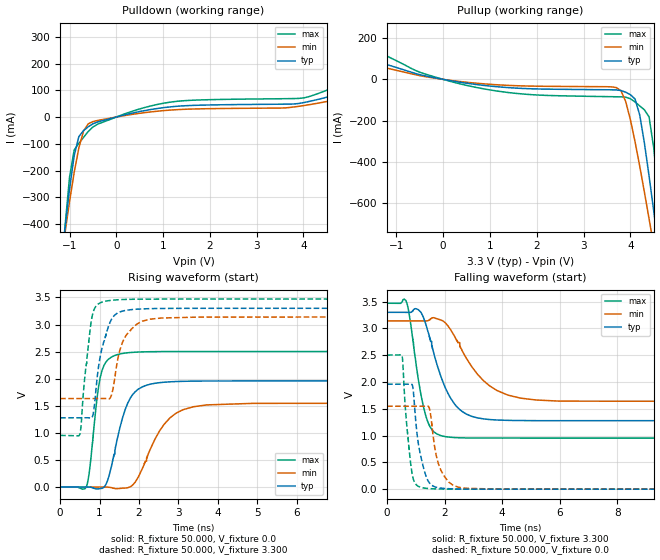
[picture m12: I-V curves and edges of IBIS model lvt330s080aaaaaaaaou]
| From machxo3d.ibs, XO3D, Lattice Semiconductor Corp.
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|   Model lvt330s080aaaaaaaaou
[Model] lvt330s080aaaaaaaaou
Model_type Output
Polarity   Non-Inverting
Enable   Active-High
Vmeas =  1.650V
Cref =  0.0F
Rref =  1.000M
Vref =  0.0V
C_comp   4.200pF   3.800pF   7.500pF
[Temperature Range]   25.000   0.105k   -40.000
[Voltage Range]   3.300V   3.140V   3.470V
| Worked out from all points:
|   slope of the pulldown table from 0 to 0.495 V, typ, clamps not added: 24.3 ohm
|   slope of the pullup table from 0 to 0.495 V, typ, clamps not added: 26.7 ohm
|   rising waveform, R_fixture 50.000, V_fixture 0.0: 20-80 % time 423ps typ, 674ps min, 236ps max; typ from 0 V to 1.96 V
|   rising waveform, R_fixture 50.000, V_fixture 3.300: 20-80 % time 301ps typ, 347ps min, 210ps max; typ from 1.28 V to 3.3 V
|   falling waveform, R_fixture 50.000, V_fixture 3.300: 20-80 % time 780ps typ, 1.19ns min, 451ps max; typ from 3.3 V to 1.28 V
|   falling waveform, R_fixture 50.000, V_fixture 0.0: 20-80 % time 315ps typ, 367ps min, 235ps max; typ from 1.96 V to 0 V
[Pulldown]
|Voltage   I(typ)   I(min)   I(max)
-3.3V     -4.507A    -3.482A    -6.263A
-1.1V     -423.3mA   -437.5mA   -416.6mA
-1V       -269.7mA   -316.9mA   -225.1mA
-900mV    -144.4mA   -206.8mA   -123.1mA
-800mV    -72.88mA   -115.2mA   -98.37mA
-700mV    -50.68mA   -52.02mA   -75.84mA
-500mV    -25.29mA   -17.01mA   -37.18mA
400mV     16.94mA    11.56mA    24.96mA
1.2V      38.8mA     26.54mA    56.81mA
4.1V      57.44mA    45.51mA    75.3mA
5.4V      124.8mA    95.07mA    178.5mA
6.6V      222.7mA    160.2mA    336.5mA
[Pullup]
|Voltage   I(typ)   I(min)   I(max)
-3.3V     151.1mA    104.7mA    247.2mA
-2.4V     144.7mA    104.5mA    232mA
600mV     -21.83mA   -16.21mA   -34.14mA
3.7V      -51.13mA   -39.8mA    -84.42mA
3.9V      -62.23mA   -107.3mA   -86.34mA
4.1V      -95.12mA   -302.3mA   -109.4mA
4.2V      -172.6mA   -421.2mA   -128.7mA
4.4V      -468.8mA   -676.6mA   -181.8mA
4.5V      -639.3mA   -809mA     -333.7mA
4.6V      -815.4mA   -943.4mA   -557.7mA
4.7V      -994.9mA   -1.079A    -803mA
6.6V      -4.562A    -3.748A    -5.893A
[Ramp]
| variable   typ   min   max
dV/dt_r   1.175/0.423n   0.929/0.671n   1.501/0.235n
dV/dt_f   1.213/0.783n   0.904/1.192n   1.510/0.451n
R_load = 50.000
[Rising Waveform]
R_fixture= 50.000
V_fixture= 0.0
V_fixture_min= 0.0
V_fixture_max= 0.0
|time   V(typ)   V(min)   V(max)
0s        17.95nV    45.29nV    212.7nV
671ps     354.9uV    -5.078uV   16.19mV
941ps     -35.03mV   100.1uV    1.669V
1.066ns   -23.85mV   409.3uV    2.159V
1.236ns   194mV      -3.367mV   2.365V
1.578ns   1.264V     -21.15mV   2.465V
1.982ns   1.806V     181.8mV    2.492V
2.787ns   1.942V     1.277V     2.501V
3.722ns   1.957V     1.516V     2.502V
20ns      1.959V     1.548V     2.502V
[Rising Waveform]
R_fixture= 50.000
V_fixture= 3.300
V_fixture_min= 3.140
V_fixture_max= 3.470
|time   V(typ)   V(min)   V(max)
0s        1.278V     1.633V     953.3mV
504ps     1.278V     1.633V     975.9mV
610ps     1.278V     1.633V     1.914V
806ps     1.281V     1.633V     3.131V
1.008ns   2.376V     1.633V     3.397V
1.22ns    2.952V     1.625V     3.44V
1.308ns   3.102V     1.706V     3.448V
1.623ns   3.255V     2.736V     3.462V
2.279ns   3.293V     3.098V     3.469V
20ns      3.3V       3.14V      3.47V
[Falling Waveform]
R_fixture= 50.000
V_fixture= 3.300
V_fixture_min= 3.140
V_fixture_max= 3.470
|time   V(typ)   V(min)   V(max)
0s        3.3V       3.14V      3.47V
653ps     3.3V       3.14V      3.522V
812ps     3.298V     3.14V      3.124V
1.087ns   3.349V     3.14V      2.049V
1.351ns   3.074V     3.138V     1.36V
1.95ns    1.989V     3.137V     988.6mV
2.758ns   1.4V       2.442V     955.8mV
3.56ns    1.299V     1.93V      953.7mV
4.633ns   1.281V     1.699V     953.3mV
20ns      1.278V     1.633V     953.2mV
[Falling Waveform]
R_fixture= 50.000
V_fixture= 0.0
V_fixture_min= 0.0
V_fixture_max= 0.0
|time   V(typ)   V(min)   V(max)
0s        1.959V     1.548V     2.502V
526ps     1.959V     1.548V     2.483V
674ps     1.959V     1.548V     1.265V
879ps     1.942V     1.548V     266.7mV
1.088ns   848.4mV    1.548V     52.75mV
1.265ns   405.2mV    1.548V     23.36mV
1.47ns    117.9mV    1.513V     10.42mV
1.871ns   19.48mV    352.3mV    2.543mV
2.489ns   3.267mV    35.24mV    311.1uV
20ns      78.12nV    217.8nV    235.9nV
